// 所有带轴和手动控制系统的基本对象（基类）
FUNCTION_BLOCK FB_Subsystem_Root
VAR_INPUT	
	// =============== 控制轴的手动按钮 =====================
	bButtonAxisFwIn		AT%I*	: BOOL;						// 正转信号(按钮)
	bButtonAxisBwIn		AT%I*	: BOOL;						// 反转信号(按钮)
END_VAR
VAR_OUTPUT
	// =============== 错误变量 ===========================
	bAxisError					: BOOL;						// 轴报错标志位
	nAxisErrorID				: UDINT;					// 轴报错ID

	// =============== 轴、按钮输出信号 ====
	bAxisMoves					: BOOL;						// 如果为TRUE，则轴正在运动
	bButtonAxisFwOut			: BOOL;						// 正转输出信号
	bButtonAxisBwOut			: BOOL;						// 反转输出信号		
END_VAR
VAR
	// =============== 停止、复位以及启动的完成信号 ======
	bHaltDone					: BOOL;						// 如果为TRUE，则停止完成
	bResetDone					: BOOL;						// 如果为TRUE，则复位完成
	bStartingDone				: BOOL;						// 如果为TRUE，则启动完成
	
	// =============== 使能信号 ===================================
	bComprAirEnabledLocal		: BOOL;						// 成功压缩（气缸）空气
	bAxisEnableLocal			: BOOL;						// 如果为TRUE，则轴使能
	bSensorEnableLocal			: BOOL;						// 启用传感器信号
	bManualAxisEnableLocal		: BOOL;						// 允许轴被手动控制
	bManualCylinderEnable		: BOOL;						// 允许气缸被手动控制

	// =============== 请求 ===========================
	bHaltRequest				: BOOL;						// 如果为TRUE，则设备接受到停止请求
	bResetRequest				: BOOL;						// 如果为TRUE，则设备接受到复位请求

	// =============== 轴 ======================================
	fbAxis						: FB_Axis;					// 轴对象
	fAxisVelo					: LREAL;					// 轴运动的设定速度
	
	// =============== 信号处理功能块 =======================
	fbButtonAxisFw				: FB_SignalHandling;	// 处理轴正转
	fbButtonAxisBw				: FB_SignalHandling;	// 处理轴反转
	
	// =============== 其他 ==========================
	fbTriggerStartingStart		: R_TRIG;					// 检测启动上升沿
	fbTriggerResetStart			: R_TRIG;					// 检测复位上升沿			
	bMoved						: BOOL;						// 如果为TRUE，则轴运动过
END_VAR

// =========================================================
;
// =========================================================

PROPERTY bState_HaltDone : BOOL
GET
bState_HaltDone := bHaltDone;
END_GET
END_PROPERTY

PROPERTY bState_ResetDone : BOOL
GET
bState_ResetDone := bResetDone;
END_GET
END_PROPERTY

PROPERTY bState_StartingDone : BOOL
GET
bState_StartingDone := bStartingDone;
END_GET
END_PROPERTY

METHOD CylicCheck
VAR_INPUT
END_VAR

// 循环检查轴的状态
fbAxis.CylicCheck();
END_METHOD

METHOD PUBLIC Enable
VAR_INPUT
	bComprAirEnabled		: BOOL;			// 压缩（气缸）空气
	bAxisEnable				: BOOL;			// 使能轴
	bSensorEnable			: BOOL;			// 启用传感器
	bManualAxisEnable		: BOOL;			// 允许手动控制轴
END_VAR
// =========================================================
// 将方法的输入传递给功能块本地

	bComprAirEnabledLocal	:= bComprAirEnabled;
	bAxisEnableLocal		:= bAxisEnable;
	bSensorEnableLocal		:= bSensorEnable;
	bManualAxisEnableLocal	:= bManualAxisEnable;
	
// =========================================================	
// 使能轴

	fbAxis.Enable(bEnable := bAxisEnableLocal);					

// =========================================================
// 手动压缩气缸空气 
		
	bManualCylinderEnable := bManualAxisEnableLocal AND bComprAirEnabledLocal;
 
// =========================================================
// 手动控制轴运动

	fbButtonAxisFw.Enable(bEnable := bManualAxisEnableLocal );
	fbButtonAxisBw.Enable(bEnable := bManualAxisEnableLocal );

	
// =========================================================
END_METHOD

PROPERTY fAxisVelocity : LREAL
GET
fAxisVelocity := fAxisVelo;
END_GET
SET
fAxisVelo := fAxisVelocity;
END_SET
END_PROPERTY

METHOD PUBLIC Halt
VAR_INPUT
	bHalt		: BOOL;				// 停止请求
END_VAR

// =========================================================
// 停止轴

	fbAxis.Halt(bDriveHalt := bHaltRequest := bHalt);

// =========================================================
// 获取停止状态

	bHaltDone := fbAxis.bState_HaltDone;

// =========================================================
END_METHOD

METHOD PUBLIC InputOutput
VAR_INPUT
END_VAR
// =========================================================
// 关联输入输出状态变量
		
	fbButtonAxisFw.SetOutput();	
	fbButtonAxisBw.SetOutput();
	
	bAxisMoves 		:= fbAxis.bMoves;
	bAxisError		:= fbAxis.bError;
	nAxisErrorID	:= fbAxis.nErrorID;
	
	
	fbButtonAxisFw( bInput:=bButtonAxisFwIn , bOut=>bButtonAxisFwOut );
	fbButtonAxisBw( bInput:=bButtonAxisBwIn , bOut=>bButtonAxisBwOut );


// =========================================================
END_METHOD

METHOD PUBLIC Manual
VAR_INPUT
END_VAR
// =========================================================
// 手动模式的轴控

// 手动控制轴运动时，重置bHaltDone，将bMove置为TRUE
IF fbButtonAxisBw.bOut OR fbButtonAxisFw.bOut THEN
    bHaltDone := FALSE;
    bMoved := TRUE;
	
	// 如果反转按钮输出信号为TRUE，反转
	IF fbButtonAxisBw.bOut THEN
		fbAxis.MoveBw();
		
	// 如果正转按钮输出信号为TRUE，正转
	ELSIF fbButtonAxisFw.bOut THEN
		fbAxis.MoveFw();
	END_IF
	
// 如果轴没有受到正反转的控制，则保持停止
ELSIF (NOT fbButtonAxisBw.bOut AND NOT fbButtonAxisFw.bOut)  THEN
		
	IF bMoved AND NOT bHaltDone THEN
		Halt(bHalt := TRUE);		
	ELSE
		Halt(bHalt := FALSE);
		bMoved := FALSE;
	END_IF
		
END_IF
// =========================================================
END_METHOD

PROPERTY R_Axis : Reference TO FB_Axis
GET
R_Axis REF= fbAxis;
END_GET
SET
fbAxis := R_Axis;
END_SET
END_PROPERTY

METHOD PUBLIC Reset
VAR_INPUT
	bReset		: BOOL;				// 复位请求
END_VAR
// =========================================================
// 重置轴状态变量

	bMoved 			:= FALSE;
	bHaltDone 		:= FALSE;
	bHaltRequest	:= FALSE;

// =========================================================
// 复位轴，检测复位请求信号，传递复位相关状态变量
						
	fbTriggerResetStart(CLK := bReset);
	
	fbAxis.Reset(bDriveReset := bResetRequest:= bReset);
	
	bResetDone := fbAxis.bState_ResetDone;

// =========================================================
END_METHOD

METHOD PROTECTED ResetState
VAR_INPUT
END_VAR
// =========================================================
// 为子类的具体子系统（输送系统和分拣系统）所预先创建的虚方法
;

// =========================================================
END_METHOD

METHOD PUBLIC Starting
VAR_INPUT
	bStarting		: BOOL;			// 启动请求
END_VAR
// =========================================================

// 检测启动请求信号
fbTriggerStartingStart(CLK := bStarting);

IF fbTriggerStartingStart.Q THEN
	
	// 关联相关信号
	bStartingDone 			:= FALSE;
	
	fbAxis.fTargetVelocity 	:= fAxisVelo;
	// 初始化时，复位相关子系统状态
	ResetState();
END_IF

// 轴使能成功也意味着启动成功
bStartingDone 			:= fbAxis.bState_Enable;


// =========================================================
END_METHOD

END_FUNCTION_BLOCK
